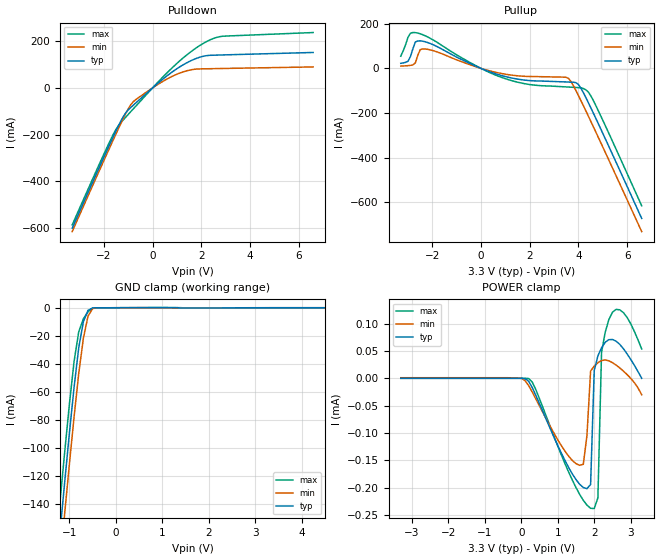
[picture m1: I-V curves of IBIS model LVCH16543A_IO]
|TEXAS INSTRUMENTS INCORPORATED
|Standard Linear and Logic Group
|IBIS Model of LVCH16543A
|16-BIT Registered Transceiver with Bus-Hold Inputs and 3-State Outputs
|TSSOP 48-pin (DGG)and SSOP 48-pin (DL) Package
[IBIS Ver]   2.1
[Comment char]  |_char
[File Name]   lvch16543a.ibs
[File Rev]   1.0
[Date]   10/9/97
[Source]   File originated at Texas Instruments, Inc.
[Notes]   The following is an IBIS list for the LVCH16543A.
|   - All test data contained in this file are derived from
|   hspice(tm) simulations.
|   - File created by Ramzi Ammar, SLL Applications
|   - This file may be incomplete or may not be fully compliant
|   with the IBIS specification. It will be replaced with a
|   version that is IBIS Revision 3.2 compliant and is complete
|   and accurate.
|   Please email all questions and comments to sllibis@ti.com.
[Disclaimer] Property of Texas Instruments Incorporated.  Unauthorized
   reproduction and/or distribution is strictly prohibited.
   This product is protected under copyright law.
" Created 1997, (C) Copyright 1997, Texas Instruments Inc.,"
   All Rights Reserved
" UNLESS THERE IS A SIGNED, WRITTEN AGREEMENT TO THE "
" CONTRARY, TEXAS INSTRUMENTS (""TI"") IS PROVIDING THE IBIS "
" MODELS ""AS IS"" AND WITHOUT ANY WARRANTY, EXPRESSED OR "
   IMPLIED.  TI assumes no liability for:
   1) the accuracy of the IBIS models provided to your
   company;
   2) the proper functioning of these IBIS models in your
   design or for any resulting applications; or
" 3) infringement of patents, copyrights or intellectual "
   property rights resulting from your use of these IBIS
   models.
   TI provides IBIS Models as a service to our customers.
" You and your company shall not distribute, sell or give "
   these models to anyone else without prior written
   permission from TI.
   TI reserves the right to make changes to our products or
   to discontinue any semiconductor product or service
" without notice, and advises our customers to obtain the "
" latest version of relevant information to verify, before "
" placing orders, that the information being relied on is "
   current.
   Please be aware that your receipt and use of the IBIS
   information provided shall serve as acceptance of these
" terms and conditions.  If you do not accept these terms,"
   you should return or destroy the IBIS models and any
   other accompanying information immediately.
[Component]   LVCH16543A_DGG
[Manufacturer]  Texas Instruments, Inc.
[Package]
|   typ   min	  max
R_pkg   0.045   0.035	  0.062
L_pkg   3.324nH   2.403nH	  5.094nH
C_pkg   0.564pF   0.341pF	  0.914nH
[Pin]	signal_name	model_name   R_pin		L_pin		C_pin
1	1OEAB   NC   0.062		5.094nH	0.856pF
2	1LEAB   NC   0.061		4.621nH	0.902pF
3	1CEAB   NC   0.06		4.316nH	0.802pF
4	GND   GND   0.059		3.968nH	0.698pF
5	1A1   LVCH16543A_IO	0.057		3.716nH	0.649pF
6	1A2   LVCH16543A_IO	0.042		3.517nH	0.652pF
7	VCC   POWER   0.041		3.16nH	0.57pF
8	1A3   LVCH16543A_IO	0.039		2.981nH	0.482pF
9	1A4   LVCH16543A_IO	0.039		2.809nH	0.447pF
10	1A5   LVCH16543A_IO	0.038		2.715nH	0.409pF
11	GND   GND   0.041		2.675nH	0.391pF
12	1A6   LVCH16543A_IO	0.039		2.536nH	0.366pF
13	1A7   LVCH16543A_IO	0.039		2.457nH	0.348pF
14	1A8   LVCH16543A_IO	0.038		2.411nH	0.353pF
15	2A1   LVCH16543A_IO	0.039		2.456nH	0.355pF
16	2A2   LVCH16543A_IO	0.039		2.471nH	0.349pF
17	2A3   LVCH16543A_IO	0.04		2.58nH	0.37pF
18	GND   GND   0.038		2.651nH	0.389pF
19	2A4   LVCH16543A_IO	0.038		2.739nH	0.411pF
20	2A5   LVCH16543A_IO	0.039		2.838nH	0.449pF
21	2A6   LVCH16543A_IO	0.038		2.988nH	0.484pF
22	VCC   POWER   0.038		3.105nH	0.564pF
23	2A7   LVCH16543A_IO	0.04		3.427nH	0.638pF
24	2A8   LVCH16543A_IO	0.056		3.654nH	0.641pF
25	GND   GND   0.057		3.932nH	0.7pF
26	2CEAB   NC   0.058		4.257nH	0.806pF
27	2LEAB   NC   0.057		4.58nH	0.914pF
28	2OEAB   NC   0.059		5.038nH	0.861pF
29	2OEBA   NC   0.06		5.058nH	0.858pF
30	2LEBA   NC   0.056		4.543nH	0.904pF
31	2CEBA   NC   0.057		4.24nH	0.803pF
32	GND   GND   0.057		3.929nH	0.7pF
33	2B8   LVCH16543A_IO	0.056		3.616nH	0.637pF
34	2B7   LVCH16543A_IO	0.037		3.368nH	0.64pF
35	VCC   POWER   0.036		3.024nH	0.563pF
36	2B6   LVCH16543A_IO	0.035		2.876nH	0.474pF
37	2B5   LVCH16543A_IO	0.035		2.745nH	0.444pF
38	2B4   LVCH16543A_IO	0.037		2.683nH	0.405pF
39	GND   GND   0.038		2.603nH	0.382pF
40	2B3   LVCH16543A_IO	0.038		2.51nH	0.362pF
41	2B2   LVCH16543A_IO	0.036		2.412nH	0.341pF
42	2B1   LVCH16543A_IO	0.038		2.416nH	0.349pF
43	1B8   LVCH16543A_IO	0.037		2.403nH	0.349pF
44	1B7   LVCH16543A_IO	0.037		2.429nH	0.341pF
45	1B6   LVCH16543A_IO	0.036		2.482nH	0.358pF
46	GND   GND   0.037		2.615nH	0.381pF
47	1B5   LVCH16543A_IO	0.035		2.669nH	0.402pF
48	1B4   LVCH16543A_IO	0.036		2.763nH	0.442pF
49	1B3   LVCH16543A_IO	0.036		2.942nH	0.478pF
50	VCC   POWER   0.035		3.053nH	0.564pF
51	1B2   LVCH16543A_IO	0.036		3.409nH	0.641pF
52	1B1   LVCH16543A_IO	0.058		3.698nH	0.641pF
53	GND   GND   0.059		3.975nH	0.697pF
54	1CEBA   NC   0.061		4.327nH	0.802pF
55	1LEBA   NC   0.061		4.624nH	0.905pF
56	1OEBA   NC   0.06		5.063nH	0.858pF
|   Component LVCH16543A_DL
[Component]   LVCH16543A_DL
[Manufacturer]  Texas Instruments, Inc.
[Package]
|   typ   min	  max
R_pkg   0.055   0.048	  0.067
L_pkg   6.539nH   4.802nH	  9.746nH
C_pkg   0.857pF   0.5pF	  1.351pF
[Pin]	signal_name	model_name   R_pin	L_pin   C_pin
1	1OEAB   NC   0.064	9.646nH	1.202pF
2	1LEAB   NC   0.059	8.723nH	1.348pF
3	1CEAB   NC   0.059	8.139nH	1.223pF
4	GND   GND   0.056	7.554nH	1.088pF
5	1A1   LVCH16543A_IO  0.054	6.991nH	0.966pF
6	1A2   LVCH16543A_IO  0.053	6.659nH	0.973pF
7	VCC   POWER   0.055	6.321nH	0.905pF
8	1A3   LVCH16543A_IO  0.055	5.942nH	0.713pF
9	1A4   LVCH16543A_IO  0.057	5.767nH	0.678pF
10	1A5   LVCH16543A_IO  0.054	5.459nH	0.631pF
11	GND   GND   0.051	5.224nH	0.638pF
12	1A6   LVCH16543A_IO  0.048	5.088nH	0.601pF
13	1A7   LVCH16543A_IO  0.05	5.021nH	0.518pF
14	1A8   LVCH16543A_IO  0.051	4.802nH	0.5pF
15	2A1   LVCH16543A_IO  0.051	4.803nH	0.5pF
16	2A2   LVCH16543A_IO  0.05	5.021nH	0.518pF
17	2A3   LVCH16543A_IO  0.048	5.088nH	0.601pF
18	GND   GND   0.051	5.224nH	0.638pF
19	2A4   LVCH16543A_IO  0.054	5.459nH	0.631pF
20	2A5   LVCH16543A_IO  0.057	5.768nH	0.677pF
21	2A6   LVCH16543A_IO  0.055	5.942nH	0.715pF
22	VCC   POWER   0.055	6.321nH	0.907pF
23	2A7   LVCH16543A_IO  0.053	6.659nH	0.972pF
24	2A8   LVCH16543A_IO  0.054	6.991nH	0.966pF
25	GND   GND   0.056	7.554nH	1.087pF
26	2CEAB   NC   0.059	8.139nH	1.223pF
27	2LEAB   NC   0.059	8.727nH	1.351pF
28	2OEAB   NC   0.067	9.746nH	1.21pF
29	2OEBA   NC   0.063	9.63nH	1.203pF
30	2LEBA   NC   0.06	8.751nH	1.349pF
31	2CEBA   NC   0.06	8.184nH	1.224pF
32	GND   GND   0.056	7.543nH	1.087pF
33	2B8   LVCH16543A_IO  0.054	7.005nH	0.969pF
34	2B7   LVCH16543A_IO  0.056	6.714nH	0.975pF
35	VCC   POWER   0.058	6.384nH	0.909pF
36	2B6   LVCH16543A_IO  0.057	5.976nH	0.717pF
37	2B5   LVCH16543A_IO  0.057	5.743nH	0.677pF
38	2B4   LVCH16543A_IO  0.055	5.469nH	0.631pF
39	GND   GND   0.055	5.328nH	0.644pF
40	2B3   LVCH16543A_IO  0.052	5.189nH	0.606pF
41	2B2   LVCH16543A_IO  0.052	5.053nH	0.519pF
42	2B1   LVCH16543A_IO  0.052	4.825nH	0.502pF
43	1B8   LVCH16543A_IO  0.054	4.896nH	0.506pF
44	1B7   LVCH16543A_IO  0.052	5.093nH	0.521pF
45	1B6   LVCH16543A_IO  0.051	5.179nH	0.608pF
46	GND   GND   0.054	5.314nH	0.645pF
47	1B5   LVCH16543A_IO  0.055	5.511nH	0.632pF
48	1B4   LVCH16543A_IO  0.057	5.77nH	0.677pF
49	1B3   LVCH16543A_IO  0.055	5.956nH	0.716pF
50	VCC   POWER   0.055	6.32nH	0.905pF
51	1B2   LVCH16543A_IO  0.052	6.621nH	0.968pF
52	1B1   LVCH16543A_IO  0.053	6.974nH	0.966pF
53	GND   GND   0.057	7.571nH	1.089pF
54	1CEBA   NC   0.057	8.097nH	1.219pF
55	1LEBA   NC   0.059	8.723nH	1.349pF
56	1OEBA   NC   0.061	9.56nH	1.199pF
| Models and submodels in the file (1): LVCH16543A_IO (I/O)
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|   Model LVCH16543A_IO
[Model]   LVCH16543A_IO
Model_type   I/O
Polarity   Inverting
Enable   Active-Low
Vinl = 0.8V
Vinh = 2.0V
|variable   typ   min   max
C_comp   7.5pF   NA   NA
[Voltage range]   3.3   3.0   3.6
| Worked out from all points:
|   slope of the pulldown table from 0 to 0.495 V, typ, clamps not added: 11.3 ohm
|   slope of the pullup table from 0 to 0.495 V, typ, clamps not added: 24.4 ohm
|   GND clamp passes 1 mA (typ) near -0.55 V on its own axis
[Pullup]   | Note: Vtable = Vcc - Voutput
|   Voltage   I(typ)   I(min)   I(max)
-3.3V     22.81mA    10.53mA    55.03mA
-3V       32.43mA    12.43mA    140.2mA
-2.7V     118.5mA    25mA       160.5mA
-2.5V     123.5mA    84.3mA     155.3mA
-2.3V     119.6mA    87.06mA    146.5mA
900mV     -33.6mA    -23.94mA   -42.25mA
2V        -54.37mA   -36.12mA   -72.22mA
3.6V      -60.99mA   -45.2mA    -83.48mA
4V        -72.16mA   -121.3mA   -85.98mA
4.3V      -129.4mA   -188.8mA   -95.53mA
4.5V      -174.3mA   -234.9mA   -121mA
6.6V      -672.3mA   -731.3mA   -615.7mA
[Pulldown]
|   Voltage   I(typ)   I(min)   I(max)
-3.3V     -601.1mA   -615.7mA   -586.9mA
-1.6V     -206mA     -219.5mA   -196.3mA
-1.2V     -122.4mA   -130.6mA   -136.6mA
-1V       -94.45mA   -89.95mA   -113.6mA
-800mV    -74.87mA   -59.87mA   -90.79mA
0V        -4.15nA    -5.398nA   -5.521nA
700mV     60.21mA    44.13mA    75.53mA
1.3V      101.8mA    70.23mA    132.3mA
1.9V      130.4mA    81.62mA    179.1mA
2.5V      140.4mA    82.79mA    212mA
2.9V      141.6mA    83.56mA    221.9mA
6.6V      152.1mA    90.13mA    237.6mA
[GND_Clamp]
|   Voltage   I(typ)   I(min)   I(max)
-3.3V     -942.5mA   -963.7mA   -921.9mA
-1.3V     -194.7mA   -217.2mA   -173mA
-1.2V     -158.9mA   -181.2mA   -137.2mA
-1.1V     -123.6mA   -145.8mA   -102.1mA
-1V       -89.12mA   -111.2mA   -68.46mA
-900mV    -56.58mA   -77.71mA   -38.16mA
-800mV    -28.41mA   -46.81mA   -17.13mA
-700mV    -9.874mA   -21.66mA   -7.854mA
-600mV    -1.846mA   -5.896mA   -2.849mA
-500mV    -110.1uA   -562.3uA   -275.2uA
0V        -4.15nA    -5.398nA   -5.475nA
6.6V      40.83nA    1.085uA    9.886nA
[POWER_Clamp]   | Note: Vtable = Vcc - Voutput
|   Voltage   I(typ)   I(min)   I(max)
-3.3V     40.83nA    1.085uA    10.35nA
200mV     -5.059uA   -13.02uA   -399.4nA
1.5V      -184.9uA   -155.8uA   -199.5uA
1.7V      -199.5uA   -157uA     -222.7uA
1.8V      -201.5uA   -104.7uA   -231.6uA
1.9V      -194uA     13.24uA    -237.4uA
2V        14.37uA    22.38uA    -237.8uA
2.1V      40.95uA    28.47uA    -218.3uA
2.2V      55.66uA    32.47uA    47.56uA
2.4V      70.58uA    32.05uA    107.1uA
2.8V      53.94uA    13.17uA    119.9uA
3.3V      -4.15nA    -30.02uA   53.61uA
[Ramp]
|Variable   typ   min   max
dV/dt_r   1.2363E+00/6.0300E-10  9.4684E-01/9.1619E-10  1.4784E+00/4.5691E-10
dV/dt_f   1.6120E+00/7.3530E-10  1.3671E+00/1.3288E-09  1.8286E+00/4.4703E-10
